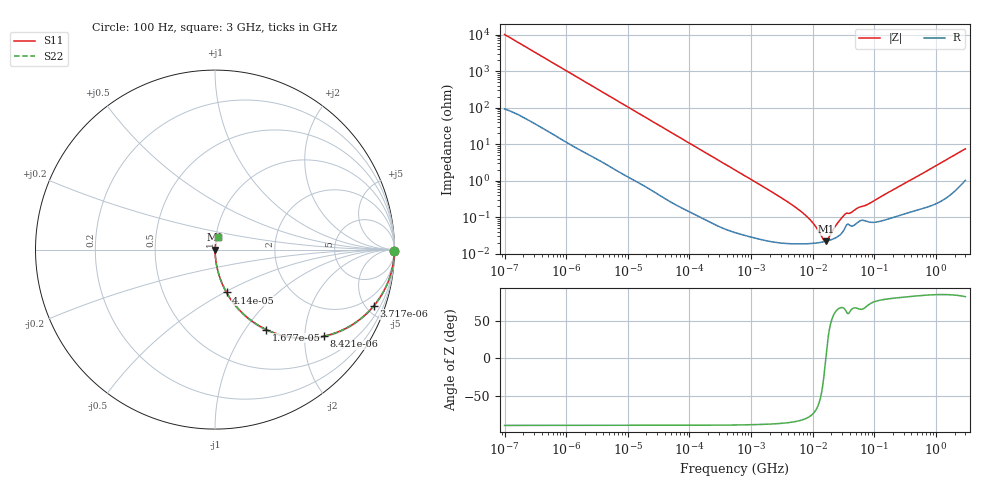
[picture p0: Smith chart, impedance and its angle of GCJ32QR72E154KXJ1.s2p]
!Murata Part Number: GCJ32QR72E154KXJ1
!These Parameters are Measured in Series Mode Connection
!Data Generated on Mar 13, 2026
!  o--ll--o
!Port1  Port2
!  o------o
!Operation Temp=25[degC], DC Bias Voltage=0[V]
!Freq. Start=100[Hz] Stop=3[GHz] 401[Steps]
# Hz S RI R 50
!Freq.(Hz) S11(Real) S11(Imag) S21(Real) S21(Imag) S12(Real) S12(Imag) S22(Real) S22(Imag)
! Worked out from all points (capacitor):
!   401 points, 100 Hz to 3 GHz, reference 50 ohm
!   read as one part in series: C = 157 nF near 109 Hz
!   lowest |Z| = 22 mohm at 16.42 MHz (marker M1)
!   series resonance near 16.27 MHz, so ESL is about 610 pH
!   S11 on the Smith chart (normalised r, x): 100 Hz: open; 3.717 kHz: 1.07, -5.60; 8.421 kHz: 1.03, -2.49; 16.77 kHz: 1.02, -1.26; 41.4 kHz: 1.01, -0.51; 3 GHz: 1.02, +0.15
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100  0.9998 -0.00987  0.000187 0.00987  0.000187 0.00987  0.9998 -0.00987
584  0.9962 -0.0566  0.00385 0.0566  0.00385 0.0566  0.9962 -0.0566
1788  0.9692 -0.1671  0.0308 0.1671  0.0308 0.1671  0.9692 -0.1671
3717  0.884 -0.3143  0.116 0.3143  0.116 0.3143  0.884 -0.3143
5476  0.7815 -0.4073  0.2185 0.4073  0.2185 0.4073  0.7815 -0.4073
8421  0.6061 -0.4827  0.3939 0.4827  0.3939 0.4827  0.6061 -0.4827
16767  0.2852 -0.4453  0.7148 0.4453  0.7148 0.4453  0.2852 -0.4453
31977  0.1017 -0.2961  0.8983 0.2961  0.8983 0.2961  0.1017 -0.2961
41399  0.0641 -0.239  0.9359 0.239  0.9359 0.239  0.0641 -0.239
121426  0.00885 -0.0871  0.9911 0.0871  0.9911 0.0871  0.00885 -0.0871
547723  0.000767 -0.0197  0.9992 0.0197  0.9992 0.0197  0.000767 -0.0197
4323298  0.000194 -0.00235  0.9998 0.00235  0.9998 0.00235  0.000194 -0.00235
6941223  0.000188 -0.00129  0.9998 0.00129  0.9998 0.00129  0.000188 -0.00129
9794414  0.000192 -0.000714  0.9998 0.000714  0.9998 0.000714  0.000192 -0.000714
1.442825e7  0.000209 -0.000162  0.9998 0.000162  0.9998 0.000162  0.000209 -0.000162
1.641694e7  0.000219 1.25e-05  0.9998 -1.25e-05  0.9998 -1.25e-05  0.000219 1.25e-05
1.789277e7  0.000228 0.00013  0.9998 -0.00013  0.9998 -0.00013  0.000228 0.00013
2.52476e7  0.000293 0.000627  0.9997 -0.000627  0.9997 -0.000627  0.000293 0.000627
3.268714e7  0.000476 0.00107  0.9995 -0.00107  0.9995 -0.00107  0.000476 0.00107
8.070971e7  0.000748 0.00219  0.9993 -0.00219  0.9993 -0.00219  0.000748 0.00219
1.751444e8  0.000938 0.00487  0.9991 -0.00487  0.9991 -0.00487  0.000938 0.00487
3e9  0.0154 0.0719  0.9846 -0.0719  0.9846 -0.0719  0.0154 0.0719
